| IBIS file stm32u595_599_5a5_5a9_wlcsp150_smps.ibs
[IBIS ver] 4.2
[File name] stm32u595_599_5a5_5a9_wlcsp150_smps.ibs
[File Rev] rev2.0
[Date]  11-09-2023
[Source] Data Created at STMicroelectronics
[Notes]  File originated from ELDO simulations.
[Disclaimer]  This information is for modeling purpose only and is
   not guaranteed. The information is subject to change without
   notice.
[Copyright] Copyright 2023 STMicroelectronics Inc.
|   Component stm32u595_599_5a5_5a9_wlcsp150_smps
[Component] stm32u595_599_5a5_5a9_wlcsp150_smps
[Manufacturer] STMicroelectronics
[Package]
| variable   typ   min   max
R_pkg  0  NA  NA
L_pkg  0  NA  NA
C_pkg  0  NA  NA
[Pin]   signal_name   model_name
A1  VDDUSB  power
A3  VDD  power
A5  PD3  io8_166m_hslv_ft
A7  PG12  io8_100m_hslv_ft
A9  PB5  io8_166m_hslv_ft
A11  VDD11 nc
A13  PE2  io8_100m_hslv_ft
AA1  VSS  gnd
AA3  PB11  io8_100m_hslv_ft
AA5  PE15  io8_100m_hslv_ft
AA7  VSS  gnd
AA9  VSS  gnd
AA11  PA5  io8_100m_ft
AA13  VDDA  nc
AB2  VDD11  nc
AB4  VDDSMPS  nc
AB6  PE14  io8_100m_hslv_ft
AB8  PE7  io8_100m_hslv_ft
AB10  PB2  io8_100m_hslv_tamp_ft
AB12  VDD  power
AC1  VDD  power
AC3  VSSSMPS  nc
AC5  VLXSMPS  nc
AC7  VDD  power
AC9  VDD  power
AC11  PC4  io8_100m_hslv_ft
AC13  VSS  gnd
B2  VDD11  nc
B4  PC11  io8_100m_hslv_ft
B6  VDD  power
B8  VDDIO2  power
B10  PB9  io8_100m_i2c_ft
B12  VDD  power
C1  PA12  io8_100m_ft
C3  VSS  gnd
C5  PD2  io8_100m_ft
C7  PG11  io8_100m_hslv_ft
C9  PB7  io8_spi_hslv_ft
C11  VSS  gnd
C13  VBAT  power
D2  PA13  io8_100m_ft
D4  PC10  io8_100m_ft
D6  VSS  gnd
D8  VSS  gnd
D10  PE3  io8_100m_hslv_tamp_ft
D12  PC13  io8_100m_ft
E1  PA11  io8_100m_ft
E3  PA10  io8_100m_usb_id
E5  PD1  io8_100m_hslv_ft
E7  PG10  io8_100m_hslv_ft
E9  PB6  io8_100m_i2c_ft
E11  PE6  io8_100m_hslv_tamp_ft
E13  PC14-OSC32_IN  nc
F2  PA9  io8_100m_usb_vbus_ft
F4  PA15  nc
F6  PD5  io8_100m_hslv_ft
F8  PG14  io8_100m_hslv_ft
F10  PE4  io8_100m_hslv_tamp_ft
F12  VSS  gnd
G1  PC8  io8_100m_ft
G3  PA8  io8_166m_hslv_ft
G5  PD0  io8_100m_hslv_ft
G7  PG13  io8_100m_hslv_ft
G9  PH3-BOOT0  nc
G11  PF0  io8_100m_hslv_ft
G13  PC15-OSC32_OUT  nc
H2  PC9  io8_100m_ft
H4  PA14  io8_100m_ft
H6  PD4  io8_100m_hslv_ft
H8  PG15  io8_100m_hslv_ft
H10  PE5  io8_100m_hslv_tamp_ft
H12  PF1  io8_100m_hslv_ft
J1  VDDIO2  power
J3  PC6  io8_100m_ft
J5  PC12  io8_166m_hslv_ft
J7  PG9  io8_100m_hslv_ft
J9  PB8  io8_100m_i2c_ft
J11  PF4  io8_spi_ft
J13  PF2  io8_100m_hslv_ft
K2  VSS  gnd
K4  PG8  io8_100m_i2c_ft
K6  PD6  io8_166m_hslv_ft
K8  PB3  io8_100m_i2c_ft
K10  PE1  io8_100m_hslv_ft
K12  PF3  io8_100m_hslv_ft
L1  PG7  io8_100m_hslv_ft
L3  PG5  io8_100m_hslv_ft
L5  PC7  io8_100m_ft
L7  PD7  io8_100m_hslv_ft
L9  PB4  io8_100m_i2c_ft
L11  PF5  io8_spi_ft
L13  VDD  power
M2  PG4  io8_100m_hslv_ft
M4  PG3  io8_100m_hslv_ft
M6  PG6  io8_100m_hslv_ft
M8  PC1  io8_spi_hslv_ft
M10  PE0  io8_100m_hslv_ft
M12  VSS  gnd
N1  PG2  io8_100m_hslv_ft
N3  PD14  io8_100m_hslv_ft
N5  PB15  nc
N7  PC5  io8_100m_tamp_ft
N9  PC0  io8_100m_hslv_ft
N11  PF6  io8_100m_hslv_ft
N13  PF7  io8_100m_hslv_ft
P2  PD15  io8_100m_hslv_ft
P4  PD11  io8_100m_hslv_ft
P6  PF13  io8_100m_hslv_ft
P8  PA4  io8_100m_hslv_ft
P10  PF8  io8_100m_hslv_ft
P12  PF9  io8_100m_hslv_ft
R1  VDD  power
R3  PD12  io8_100m_hslv_ft
R5  PB13  io8_100m_i2c_ft
R7  PF11  io8_166m_hslv_ft
R9  PA2  io8_100m_hslv_ft
R11  PF10  io8_166m_hslv_ft
R13  PH0-OSC_IN   nc
T2  VSS  gnd
T4  PB14  io8_100m_i2c_ft
T6  PG0  io8_100m_hslv_ft
T8  PB0  io8_100m_hslv_ft
T10  PA0  io8_100m_hslv_tamp_ft
T12  NRST  nc
U1  PD13  io8_100m_hslv_ft
U3  PD10  io8_100m_hslv_ft
U5  PE9  io8_166m_hslv_ft
U7  PF14  io8_100m_hslv_ft
U9  PA6  io8_100m_hslv_ft
U11  PC3  io8_100m_hslv_ft
U13  PH1-OSC_OUT  nc
V2  PD9  io8_100m_hslv_ft
V4  PE12  io8_100m_hslv_ft
V6  PE8  io8_100m_hslv_ft
V8  PF12  io8_100m_hslv_ft
V10  PA3  io8_166m_hslv_ft
V12  PC2  io8_100m_hslv_ft
W1  PD8  io8_100m_hslv_ft
W3  PB10  io8_spi_hslv_ft
W5  PE11  io8_100m_hslv_ft
W7  PG1  io8_100m_hslv_ft
W9  PB1  io8_100m_hslv_ft
W11  PA1  io8_100m_hslv_tamp_ft
W13  VSSA_VREFM  nc
Y2  PB12  io8_166m_hslv_ft
Y4  PE13  io8_100m_hslv_ft
Y6  PE10  io8_166m_hslv_ft
Y8  PF15  io8_100m_hslv_ft
Y10  PA7  io8_100m_hslv_ft
Y12  VREFP  nc
[Package Model]   481-wlcsp-150-1rdl-nodsi-220909
[Pin Mapping]   pulldown_ref   pullup_ref   | Comment
A1  nc  vddusb
A3  nc  vddiom
A5  gndio  vddiom
A7  gndio  vddiom  | Depending on IO usage
| A7  gndio  vddio2  | Depending on IO usage
A9  gndio  vddiom
A11  nc  nc
A13  gndio  vddiom
AA1  gndio  nc
AA3  gndio  vddiom
AA5  gndio  vddiom
AA7  gndio  nc
AA9  gndio  nc
AA11  gndio  vddiom
AA13  nc  nc
AB2  nc  nc
AB4  nc  nc
AB6  gndio  vddiom
AB8  gndio  vddiom
AB10  gndio  vddiom
AB12  nc  vddiom
AC1  nc  vddiom
AC3  nc  nc
AC5  nc  nc
AC7  nc  vddiom
AC9  nc  vddiom
AC11  gndio  vddiom
AC13  gndio  nc
B2  nc  nc
B4  gndio  vddiom
B6  nc  vddiom
B8  nc  vddio2
B10  gndio  vddiom
B12  nc  vddiom
C1  gndio  vddiom  | Depending on IO usage
| C1  gndio  vddusb  | Depending on IO usage
C3  gndio  nc
C5  gndio  vddiom
C7  gndio  vddiom  | Depending on IO usage
| C7  gndio  vddio2  | Depending on IO usage
C9  gndio  vddiom
C11  gndio  nc
C13  nc  vsw
D2  gndio  vddiom  | Depending on IO usage
| D2  gndio  vddusb  | Depending on IO usage
D4  gndio  vddiom
D6  gndio  nc
D8  gndio  nc
D10  gndio  vddiom
D12  gndio  vddiom  | Depending on IO usage
| D12  gndio  vsw  | Depending on IO usage
E1  gndio  vddiom  | Depending on IO usage
| E1  gndio  vddusb  | Depending on IO usage
E3  gndio  vddiom  | Depending on IO usage
| E3  gndio  vddusb  | Depending on IO usage
E5  gndio  vddiom
E7  gndio  vddiom  | Depending on IO usage
| E7  gndio  vddio2  | Depending on IO usage
E9  gndio  vddiom
E11  gndio  vddiom
E13  nc  nc
F2  gndio  vddiom  | Depending on IO usage
| F2  gndio  vddusb  | Depending on IO usage
F4  nc  nc
F6  gndio  vddiom
F8  gndio  vddiom  | Depending on IO usage
| F8  gndio  vddio2  | Depending on IO usage
F10  gndio  vddiom
F12  gndio  nc
G1  gndio  vddiom
G3  gndio  vddiom
G5  gndio  vddiom
G7  gndio  vddiom  | Depending on IO usage
| G7  gndio  vddio2  | Depending on IO usage
G9  nc  nc
G11  gndio  vddiom
G13  nc  nc
H2  gndio  vddiom
H4  gndio  vddiom
H6  gndio  vddiom
H8  gndio  vddiom  | Depending on IO usage
| H8  gndio  vddio2  | Depending on IO usage
H10  gndio  vddiom
H12  gndio  vddiom
J1  nc  vddio2
J3  gndio  vddiom
J5  gndio  vddiom
J7  gndio  vddiom  | Depending on IO usage
| J7  gndio  vddio2  | Depending on IO usage
J9  gndio  vddiom
J11  gndio  vddiom
J13  gndio  vddiom
K2  gndio  nc
K4  gndio  vddiom  | Depending on IO usage
| K4  gndio  vddio2  | Depending on IO usage
K6  gndio  vddiom
K8  gndio  vddiom
K10  gndio  vddiom
K12  gndio  vddiom
L1  gndio  vddiom  | Depending on IO usage
| L1  gndio  vddio2  | Depending on IO usage
L3  gndio  vddiom  | Depending on IO usage
| L3  gndio  vddio2  | Depending on IO usage
L5  gndio  vddiom
L7  gndio  vddiom
L9  gndio  vddiom
L11  gndio  vddiom
L13  nc  vddiom
M2  gndio  vddiom  | Depending on IO usage
| M2  gndio  vddio2  | Depending on IO usage
M4  gndio  vddiom  | Depending on IO usage
| M4  gndio  vddio2  | Depending on IO usage
M6  gndio  vddiom  | Depending on IO usage
| M6  gndio  vddio2  | Depending on IO usage
M8  gndio  vddiom
M10  gndio  vddiom
M12  gndio  nc
N1  gndio  vddiom  | Depending on IO usage
| N1  gndio  vddio2  | Depending on IO usage
N3  gndio  vddiom
N5  nc  nc
N7  gndio  vddiom
N9  gndio  vddiom
N11  gndio  vddiom
N13  gndio  vddiom
P2  gndio  vddiom
P4  gndio  vddiom
P6  gndio  vddiom
P8  gndio  vddiom
P10  gndio  vddiom
P12  gndio  vddiom
R1  nc  vddiom
R3  gndio  vddiom
R5  gndio  vddiom
R7  gndio  vddiom
R9  gndio  vddiom
R11  gndio  vddiom
R13  nc  nc
T2  gndio  nc
T4  gndio  vddiom
T6  gndio  vddiom
T8  gndio  vddiom
T10  gndio  vddiom
T12  nc  nc
U1  gndio  vddiom
U3  gndio  vddiom
U5  gndio  vddiom
U7  gndio  vddiom
U9  gndio  vddiom
U11  gndio  vddiom
U13  nc  nc
V2  gndio  vddiom
V4  gndio  vddiom
V6  gndio  vddiom
V8  gndio  vddiom
V10  gndio  vddiom
V12  gndio  vddiom
W1  gndio  vddiom
W3  gndio  vddiom
W5  gndio  vddiom
W7  gndio  vddiom
W9  gndio  vddiom
W11  gndio  vddiom
W13  nc  nc
Y2  gndio  vddiom
Y4  gndio  vddiom
Y6  gndio  vddiom
Y8  gndio  vddiom
Y10  gndio  vddiom
Y12  nc  nc
[Model Selector] io8_100m_ft
io8_100m_ft_hs_1v2  "IO8_FT 100MHz high speed @ 1.2V"
io8_100m_ft_fs_1v2  "IO8_FT 100MHz fast speed @ 1.2V"
io8_100m_ft_fs_pd_1v2  "IO8_FT 100MHz fast speed @ 1.2V pulldown"
io8_100m_ft_ms_1v2  "IO8_FT 100MHz med speed @ 1.2V"
io8_100m_ft_ms_pd_1v2  "IO8_FT 100MHz med speed @ 1.2V pulldown"
io8_100m_ft_ls_1v2  "IO8_FT 100MHz low speed @ 1.2V"
io8_100m_ft_ls_pd_1v2  "IO8_FT 100MHz low speed @ 1.2V pulldown"
io8_100m_ft_hs_1v8  "IO8_FT 100MHz high speed @ 1.8V"
io8_100m_ft_hs_pd_1v8  "IO8_FT 100MHz high speed @ 1.8V pulldown"
io8_100m_ft_fs_1v8  "IO8_FT 100MHz fast speed @ 1.8V"
io8_100m_ft_fs_pd_1v8  "IO8_FT 100MHz fast speed @ 1.8V pulldown"
io8_100m_ft_ms_1v8  "IO8_FT 100MHz med speed @ 1.8V"
io8_100m_ft_ms_pd_1v8  "IO8_FT 100MHz med speed @ 1.8V pulldown"
io8_100m_ft_ls_1v8  "IO8_FT 100MHz low speed @ 1.8V"
io8_100m_ft_ls_pd_1v8  "IO8_FT 100MHz low speed @ 1.8V pulldown"
io8_100m_ft_hs_3v3  "IO8_FT 100MHz high speed @ 3.3V"
io8_100m_ft_hs_pd_3v3  "IO8_FT 100MHz high speed @ 3.3V pulldown"
io8_100m_ft_fs_3v3  "IO8_FT 100MHz fast speed @ 3.3V"
io8_100m_ft_fs_pd_3v3  "IO8_FT 100MHz fast speed @ 3.3V pulldown"
io8_100m_ft_ms_3v3  "IO8_FT 100MHz med speed @ 3.3V"
io8_100m_ft_ms_pd_3v3  "IO8_FT 100MHz med speed @ 3.3V pulldown"
io8_100m_ft_ls_3v3  "IO8_FT 100MHz low speed @ 3.3V"
io8_100m_ft_ls_pd_3v3  "IO8_FT 100MHz low speed @ 3.3V pulldown"
[Model Selector] io8_100m_hslv_ft
io8_100m_ft_hs_1v2  "IO8_FT 100MHz high speed @ 1.2V"
io8_100m_ft_hs_pu_1v2  "IO8_FT 100MHz high speed @ 1.2V pullup"
io8_100m_ft_hs_pd_1v2  "IO8_FT 100MHz high speed @ 1.2V pulldown"
io8_100m_ft_fs_1v2  "IO8_FT 100MHz fast speed @ 1.2V"
io8_100m_ft_fs_pu_1v2  "IO8_FT 100MHz fast speed @ 1.2V pullup"
io8_100m_ft_fs_pd_1v2  "IO8_FT 100MHz fast speed @ 1.2V pulldown"
io8_100m_ft_ms_1v2  "IO8_FT 100MHz med speed @ 1.2V"
io8_100m_ft_ms_pu_1v2  "IO8_FT 100MHz med speed @ 1.2V pullup"
io8_100m_ft_ms_pd_1v2  "IO8_FT 100MHz med speed @ 1.2V pulldown"
io8_100m_ft_ls_1v2  "IO8_FT 100MHz low speed @ 1.2V"
io8_100m_ft_ls_pu_1v2  "IO8_FT 100MHz low speed @ 1.2V pullup"
io8_100m_ft_ls_pd_1v2  "IO8_FT 100MHz low speed @ 1.2V pulldown"
io8_100m_ft_hs_1v8  "IO8_FT 100MHz high speed @ 1.8V"
io8_100m_ft_hs_pu_1v8  "IO8_FT 100MHz high speed @ 1.8V pullup"
io8_100m_ft_hs_pd_1v8  "IO8_FT 100MHz high speed @ 1.8V pulldown"
io8_100m_ft_fs_1v8  "IO8_FT 100MHz fast speed @ 1.8V"
io8_100m_ft_fs_pu_1v8  "IO8_FT 100MHz fast speed @ 1.8V pullup"
io8_100m_ft_fs_pd_1v8  "IO8_FT 100MHz fast speed @ 1.8V pulldown"
io8_100m_ft_ms_1v8  "IO8_FT 100MHz med speed @ 1.8V"
io8_100m_ft_ms_pu_1v8  "IO8_FT 100MHz med speed @ 1.8V pullup"
io8_100m_ft_ms_pd_1v8  "IO8_FT 100MHz med speed @ 1.8V pulldown"
io8_100m_ft_ls_1v8  "IO8_FT 100MHz low speed @ 1.8V"
io8_100m_ft_ls_pu_1v8  "IO8_FT 100MHz low speed @ 1.8V pullup"
io8_100m_ft_ls_pd_1v8  "IO8_FT 100MHz low speed @ 1.8V pulldown"
io8_100m_ft_hs_3v3  "IO8_FT 100MHz high speed @ 3.3V"
io8_100m_ft_hs_pu_3v3  "IO8_FT 100MHz high speed @ 3.3V pullup"
io8_100m_ft_hs_pd_3v3  "IO8_FT 100MHz high speed @ 3.3V pulldown"
io8_100m_ft_fs_3v3  "IO8_FT 100MHz fast speed @ 3.3V"
io8_100m_ft_fs_pu_3v3  "IO8_FT 100MHz fast speed @ 3.3V pullup"
io8_100m_ft_fs_pd_3v3  "IO8_FT 100MHz fast speed @ 3.3V pulldown"
io8_100m_ft_ms_3v3  "IO8_FT 100MHz med speed @ 3.3V"
io8_100m_ft_ms_pu_3v3  "IO8_FT 100MHz med speed @ 3.3V pullup"
io8_100m_ft_ms_pd_3v3  "IO8_FT 100MHz med speed @ 3.3V pulldown"
io8_100m_ft_ls_3v3  "IO8_FT 100MHz low speed @ 3.3V"
io8_100m_ft_ls_pu_3v3  "IO8_FT 100MHz low speed @ 3.3V pullup"
io8_100m_ft_ls_pd_3v3  "IO8_FT 100MHz low speed @ 3.3V pulldown"
io8_100m_hslv_ft_hs_1v2  "IO8_FT 100MHz HSLV high speed @ 1.2V"
io8_100m_hslv_ft_hs_pu_1v2  "IO8_FT 100MHz HSLV high speed @ 1.2V pullup"
io8_100m_hslv_ft_hs_pd_1v2  "IO8_FT 100MHz HSLV high speed @ 1.2V pulldown"
io8_100m_hslv_ft_fs_1v2  "IO8_FT 100MHz HSLV fast speed @ 1.2V"
io8_100m_hslv_ft_fs_pu_1v2  "IO8_FT 100MHz HSLV fast speed @ 1.2V pullup"
io8_100m_hslv_ft_fs_pd_1v2  "IO8_FT 100MHz HSLV fast speed @ 1.2V pulldown"
io8_100m_hslv_ft_ms_1v2  "IO8_FT 100MHz HSLV med speed @ 1.2V"
io8_100m_hslv_ft_ms_pu_1v2  "IO8_FT 100MHz HSLV med speed @ 1.2V pullup"
io8_100m_hslv_ft_ms_pd_1v2  "IO8_FT 100MHz HSLV med speed @ 1.2V pulldown"
io8_100m_hslv_ft_ls_1v2  "IO8_FT 100MHz HSLV low speed @ 1.2V"
io8_100m_hslv_ft_ls_pu_1v2  "IO8_FT 100MHz HSLV low speed @ 1.2V pullup"
io8_100m_hslv_ft_ls_pd_1v2  "IO8_FT 100MHz HSLV low speed @ 1.2V pulldown"
io8_100m_hslv_ft_hs_1v8  "IO8_FT 100MHz HSLV high speed @ 1.8V"
io8_100m_hslv_ft_hs_pu_1v8  "IO8_FT 100MHz HSLV high speed @ 1.8V pullup"
io8_100m_hslv_ft_hs_pd_1v8  "IO8_FT 100MHz HSLV high speed @ 1.8V pulldown"
io8_100m_hslv_ft_fs_1v8  "IO8_FT 100MHz HSLV fast speed @ 1.8V"
io8_100m_hslv_ft_fs_pu_1v8  "IO8_FT 100MHz HSLV fast speed @ 1.8V pullup"
io8_100m_hslv_ft_fs_pd_1v8  "IO8_FT 100MHz HSLV fast speed @ 1.8V pulldown"
io8_100m_hslv_ft_ms_1v8  "IO8_FT 100MHz HSLV med speed @ 1.8V"
io8_100m_hslv_ft_ms_pu_1v8  "IO8_FT 100MHz HSLV med speed @ 1.8V pullup"
io8_100m_hslv_ft_ms_pd_1v8  "IO8_FT 100MHz HSLV med speed @ 1.8V pulldown"
io8_100m_hslv_ft_ls_1v8  "IO8_FT 100MHz HSLV low speed @ 1.8V"
io8_100m_hslv_ft_ls_pu_1v8  "IO8_FT 100MHz HSLV low speed @ 1.8V pullup"
io8_100m_hslv_ft_ls_pd_1v8  "IO8_FT 100MHz HSLV low speed @ 1.8V pulldown"
io8_100m_hslv_ft_hs_2v5  "IO8_FT 100MHz HSLV high speed @ 2.5V"
io8_100m_hslv_ft_hs_pu_2v5  "IO8_FT 100MHz HSLV high speed @ 2.5V pullup"
io8_100m_hslv_ft_hs_pd_2v5  "IO8_FT 100MHz HSLV high speed @ 2.5V pulldown"
io8_100m_hslv_ft_fs_2v5  "IO8_FT 100MHz HSLV fast speed @ 2.5V"
io8_100m_hslv_ft_fs_pu_2v5  "IO8_FT 100MHz HSLV fast speed @ 2.5V pullup"
io8_100m_hslv_ft_fs_pd_2v5  "IO8_FT 100MHz HSLV fast speed @ 2.5V pulldown"
io8_100m_hslv_ft_ms_2v5  "IO8_FT 100MHz HSLV med speed @ 2.5V"
io8_100m_hslv_ft_ms_pu_2v5  "IO8_FT 100MHz HSLV med speed @ 2.5V pullup"
io8_100m_hslv_ft_ms_pd_2v5  "IO8_FT 100MHz HSLV med speed @ 2.5V pulldown"
io8_100m_hslv_ft_ls_2v5  "IO8_FT 100MHz HSLV low speed @ 2.5V"
io8_100m_hslv_ft_ls_pu_2v5  "IO8_FT 100MHz HSLV low speed @ 2.5V pullup"
io8_100m_hslv_ft_ls_pd_2v5  "IO8_FT 100MHz HSLV low speed @ 2.5V pulldown"
[Model Selector] io8_100m_hslv_tamp_ft
io8_100m_ft_hs_1v2  "IO8_FT 100MHz high speed @ 1.2V"
io8_100m_ft_hs_pu_1v2  "IO8_FT 100MHz high speed @ 1.2V pullup"
io8_100m_ft_hs_pd_1v2  "IO8_FT 100MHz high speed @ 1.2V pulldown"
io8_100m_ft_fs_1v2  "IO8_FT 100MHz fast speed @ 1.2V"
io8_100m_ft_fs_pu_1v2  "IO8_FT 100MHz fast speed @ 1.2V pullup"
io8_100m_ft_fs_pd_1v2  "IO8_FT 100MHz fast speed @ 1.2V pulldown"
io8_100m_ft_ms_1v2  "IO8_FT 100MHz med speed @ 1.2V"
io8_100m_ft_ms_pu_1v2  "IO8_FT 100MHz med speed @ 1.2V pullup"
io8_100m_ft_ms_pd_1v2  "IO8_FT 100MHz med speed @ 1.2V pulldown"
io8_100m_ft_ls_1v2  "IO8_FT 100MHz low speed @ 1.2V"
io8_100m_ft_ls_pu_1v2  "IO8_FT 100MHz low speed @ 1.2V pullup"
io8_100m_ft_ls_pd_1v2  "IO8_FT 100MHz low speed @ 1.2V pulldown"
io8_100m_ft_hs_1v8  "IO8_FT 100MHz high speed @ 1.8V"
io8_100m_ft_hs_pu_1v8  "IO8_FT 100MHz high speed @ 1.8V pullup"
io8_100m_ft_hs_pd_1v8  "IO8_FT 100MHz high speed @ 1.8V pulldown"
io8_100m_ft_fs_1v8  "IO8_FT 100MHz fast speed @ 1.8V"
io8_100m_ft_fs_pu_1v8  "IO8_FT 100MHz fast speed @ 1.8V pullup"
io8_100m_ft_fs_pd_1v8  "IO8_FT 100MHz fast speed @ 1.8V pulldown"
io8_100m_ft_ms_1v8  "IO8_FT 100MHz med speed @ 1.8V"
io8_100m_ft_ms_pu_1v8  "IO8_FT 100MHz med speed @ 1.8V pullup"
io8_100m_ft_ms_pd_1v8  "IO8_FT 100MHz med speed @ 1.8V pulldown"
io8_100m_ft_ls_1v8  "IO8_FT 100MHz low speed @ 1.8V"
io8_100m_ft_ls_pu_1v8  "IO8_FT 100MHz low speed @ 1.8V pullup"
io8_100m_ft_ls_pd_1v8  "IO8_FT 100MHz low speed @ 1.8V pulldown"
io8_100m_ft_hs_3v3  "IO8_FT 100MHz high speed @ 3.3V"
io8_100m_ft_hs_pu_3v3  "IO8_FT 100MHz high speed @ 3.3V pullup"
io8_100m_ft_hs_pd_3v3  "IO8_FT 100MHz high speed @ 3.3V pulldown"
io8_100m_ft_fs_3v3  "IO8_FT 100MHz fast speed @ 3.3V"
io8_100m_ft_fs_pu_3v3  "IO8_FT 100MHz fast speed @ 3.3V pullup"
io8_100m_ft_fs_pd_3v3  "IO8_FT 100MHz fast speed @ 3.3V pulldown"
io8_100m_ft_ms_3v3  "IO8_FT 100MHz med speed @ 3.3V"
io8_100m_ft_ms_pu_3v3  "IO8_FT 100MHz med speed @ 3.3V pullup"
io8_100m_ft_ms_pd_3v3  "IO8_FT 100MHz med speed @ 3.3V pulldown"
io8_100m_ft_ls_3v3  "IO8_FT 100MHz low speed @ 3.3V"
io8_100m_ft_ls_pu_3v3  "IO8_FT 100MHz low speed @ 3.3V pullup"
io8_100m_ft_ls_pd_3v3  "IO8_FT 100MHz low speed @ 3.3V pulldown"
io8_100m_hslv_ft_hs_1v2  "IO8_FT 100MHz HSLV high speed @ 1.2V"
io8_100m_hslv_ft_hs_pu_1v2  "IO8_FT 100MHz HSLV high speed @ 1.2V pullup"
io8_100m_hslv_ft_hs_pd_1v2  "IO8_FT 100MHz HSLV high speed @ 1.2V pulldown"
io8_100m_hslv_ft_fs_1v2  "IO8_FT 100MHz HSLV fast speed @ 1.2V"
io8_100m_hslv_ft_fs_pu_1v2  "IO8_FT 100MHz HSLV fast speed @ 1.2V pullup"
io8_100m_hslv_ft_fs_pd_1v2  "IO8_FT 100MHz HSLV fast speed @ 1.2V pulldown"
io8_100m_hslv_ft_ms_1v2  "IO8_FT 100MHz HSLV med speed @ 1.2V"
io8_100m_hslv_ft_ms_pu_1v2  "IO8_FT 100MHz HSLV med speed @ 1.2V pullup"
io8_100m_hslv_ft_ms_pd_1v2  "IO8_FT 100MHz HSLV med speed @ 1.2V pulldown"
io8_100m_hslv_ft_ls_1v2  "IO8_FT 100MHz HSLV low speed @ 1.2V"
io8_100m_hslv_ft_ls_pu_1v2  "IO8_FT 100MHz HSLV low speed @ 1.2V pullup"
io8_100m_hslv_ft_ls_pd_1v2  "IO8_FT 100MHz HSLV low speed @ 1.2V pulldown"
io8_100m_hslv_ft_hs_1v8  "IO8_FT 100MHz HSLV high speed @ 1.8V"
io8_100m_hslv_ft_hs_pu_1v8  "IO8_FT 100MHz HSLV high speed @ 1.8V pullup"
io8_100m_hslv_ft_hs_pd_1v8  "IO8_FT 100MHz HSLV high speed @ 1.8V pulldown"
io8_100m_hslv_ft_fs_1v8  "IO8_FT 100MHz HSLV fast speed @ 1.8V"
io8_100m_hslv_ft_fs_pu_1v8  "IO8_FT 100MHz HSLV fast speed @ 1.8V pullup"
io8_100m_hslv_ft_fs_pd_1v8  "IO8_FT 100MHz HSLV fast speed @ 1.8V pulldown"
io8_100m_hslv_ft_ms_1v8  "IO8_FT 100MHz HSLV med speed @ 1.8V"
io8_100m_hslv_ft_ms_pu_1v8  "IO8_FT 100MHz HSLV med speed @ 1.8V pullup"
io8_100m_hslv_ft_ms_pd_1v8  "IO8_FT 100MHz HSLV med speed @ 1.8V pulldown"
io8_100m_hslv_ft_ls_1v8  "IO8_FT 100MHz HSLV low speed @ 1.8V"
io8_100m_hslv_ft_ls_pu_1v8  "IO8_FT 100MHz HSLV low speed @ 1.8V pullup"
io8_100m_hslv_ft_ls_pd_1v8  "IO8_FT 100MHz HSLV low speed @ 1.8V pulldown"
io8_100m_hslv_ft_hs_2v5  "IO8_FT 100MHz HSLV high speed @ 2.5V"
io8_100m_hslv_ft_hs_pu_2v5  "IO8_FT 100MHz HSLV high speed @ 2.5V pullup"
io8_100m_hslv_ft_hs_pd_2v5  "IO8_FT 100MHz HSLV high speed @ 2.5V pulldown"
io8_100m_hslv_ft_fs_2v5  "IO8_FT 100MHz HSLV fast speed @ 2.5V"
io8_100m_hslv_ft_fs_pu_2v5  "IO8_FT 100MHz HSLV fast speed @ 2.5V pullup"
io8_100m_hslv_ft_fs_pd_2v5  "IO8_FT 100MHz HSLV fast speed @ 2.5V pulldown"
io8_100m_hslv_ft_ms_2v5  "IO8_FT 100MHz HSLV med speed @ 2.5V"
io8_100m_hslv_ft_ms_pu_2v5  "IO8_FT 100MHz HSLV med speed @ 2.5V pullup"
io8_100m_hslv_ft_ms_pd_2v5  "IO8_FT 100MHz HSLV med speed @ 2.5V pulldown"
io8_100m_hslv_ft_ls_2v5  "IO8_FT 100MHz HSLV low speed @ 2.5V"
io8_100m_hslv_ft_ls_pu_2v5  "IO8_FT 100MHz HSLV low speed @ 2.5V pullup"
io8_100m_hslv_ft_ls_pd_2v5  "IO8_FT 100MHz HSLV low speed @ 2.5V pulldown"
io8_ft_v33_hs_1v2  "IO8_FT_V33 high speed @ 1.2V"
io8_ft_v33_hs_pu_1v2  "IO8_FT_V33 high speed @ 1.2V pullup"
io8_ft_v33_hs_pd_1v2  "IO8_FT_V33 high speed @ 1.2V pulldown"
io8_ft_v33_fs_1v2  "IO8_FT_V33 fast speed @ 1.2V"
io8_ft_v33_fs_pu_1v2  "IO8_FT_V33 fast speed @ 1.2V pullup"
io8_ft_v33_fs_pd_1v2  "IO8_FT_V33 fast speed @ 1.2V pulldown"
io8_ft_v33_ms_1v2  "IO8_FT_V33 med speed @ 1.2V"
io8_ft_v33_ms_pu_1v2  "IO8_FT_V33 med speed @ 1.2V pullup"
io8_ft_v33_ms_pd_1v2  "IO8_FT_V33 med speed @ 1.2V pulldown"
io8_ft_v33_ls_1v2  "IO8_FT_V33 low speed @ 1.2V"
io8_ft_v33_ls_pu_1v2  "IO8_FT_V33 low speed @ 1.2V pullup"
io8_ft_v33_ls_pd_1v2  "IO8_FT_V33 low speed @ 1.2V pulldown"
io8_ft_v33_hs_1v8  "IO8_FT_V33 high speed @ 1.8V"
io8_ft_v33_hs_pu_1v8  "IO8_FT_V33 high speed @ 1.8V pullup"
io8_ft_v33_hs_pd_1v8  "IO8_FT_V33 high speed @ 1.8V pulldown"
io8_ft_v33_fs_1v8  "IO8_FT_V33 fast speed @ 1.8V"
io8_ft_v33_fs_pu_1v8  "IO8_FT_V33 fast speed @ 1.8V pullup"
io8_ft_v33_fs_pd_1v8  "IO8_FT_V33 fast speed @ 1.8V pulldown"
io8_ft_v33_ms_1v8  "IO8_FT_V33 med speed @ 1.8V"
io8_ft_v33_ms_pu_1v8  "IO8_FT_V33 med speed @ 1.8V pullup"
io8_ft_v33_ms_pd_1v8  "IO8_FT_V33 med speed @ 1.8V pulldown"
io8_ft_v33_ls_1v8  "IO8_FT_V33 low speed @ 1.8V"
io8_ft_v33_ls_pu_1v8  "IO8_FT_V33 low speed @ 1.8V pullup"
io8_ft_v33_ls_pd_1v8  "IO8_FT_V33 low speed @ 1.8V pulldown"
io8_ft_v33_hs_3v3  "IO8_FT_V33 high speed @ 3.3V"
io8_ft_v33_hs_pu_3v3  "IO8_FT_V33 high speed @ 3.3V pullup"
io8_ft_v33_hs_pd_3v3  "IO8_FT_V33 high speed @ 3.3V pulldown"
io8_ft_v33_fs_3v3  "IO8_FT_V33 fast speed @ 3.3V"
io8_ft_v33_fs_pu_3v3  "IO8_FT_V33 fast speed @ 3.3V pullup"
io8_ft_v33_fs_pd_3v3  "IO8_FT_V33 fast speed @ 3.3V pulldown"
io8_ft_v33_ms_3v3  "IO8_FT_V33 med speed @ 3.3V"
io8_ft_v33_ms_pu_3v3  "IO8_FT_V33 med speed @ 3.3V pullup"
io8_ft_v33_ms_pd_3v3  "IO8_FT_V33 med speed @ 3.3V pulldown"
io8_ft_v33_ls_3v3  "IO8_FT_V33 low speed @ 3.3V"
io8_ft_v33_ls_pu_3v3  "IO8_FT_V33 low speed @ 3.3V pullup"
io8_ft_v33_ls_pd_3v3  "IO8_FT_V33 low speed @ 3.3V pulldown"
[Model Selector] io8_100m_i2c_ft
io8_100m_ft_hs_1v2  "IO8_FT 100MHz high speed @ 1.2V"
io8_100m_ft_hs_pu_1v2  "IO8_FT 100MHz high speed @ 1.2V pullup"
io8_100m_ft_hs_pd_1v2  "IO8_FT 100MHz high speed @ 1.2V pulldown"
io8_100m_ft_fs_1v2  "IO8_FT 100MHz fast speed @ 1.2V"
io8_100m_ft_fs_pu_1v2  "IO8_FT 100MHz fast speed @ 1.2V pullup"
io8_100m_ft_fs_pd_1v2  "IO8_FT 100MHz fast speed @ 1.2V pulldown"
io8_100m_ft_ms_1v2  "IO8_FT 100MHz med speed @ 1.2V"
io8_100m_ft_ms_pu_1v2  "IO8_FT 100MHz med speed @ 1.2V pullup"
io8_100m_ft_ms_pd_1v2  "IO8_FT 100MHz med speed @ 1.2V pulldown"
io8_100m_ft_ls_1v2  "IO8_FT 100MHz low speed @ 1.2V"
io8_100m_ft_ls_pu_1v2  "IO8_FT 100MHz low speed @ 1.2V pullup"
io8_100m_ft_ls_pd_1v2  "IO8_FT 100MHz low speed @ 1.2V pulldown"
io8_100m_ft_hs_1v8  "IO8_FT 100MHz high speed @ 1.8V"
io8_100m_ft_hs_pu_1v8  "IO8_FT 100MHz high speed @ 1.8V pullup"
io8_100m_ft_hs_pd_1v8  "IO8_FT 100MHz high speed @ 1.8V pulldown"
io8_100m_ft_fs_1v8  "IO8_FT 100MHz fast speed @ 1.8V"
io8_100m_ft_fs_pu_1v8  "IO8_FT 100MHz fast speed @ 1.8V pullup"
io8_100m_ft_fs_pd_1v8  "IO8_FT 100MHz fast speed @ 1.8V pulldown"
io8_100m_ft_ms_1v8  "IO8_FT 100MHz med speed @ 1.8V"
io8_100m_ft_ms_pu_1v8  "IO8_FT 100MHz med speed @ 1.8V pullup"
io8_100m_ft_ms_pd_1v8  "IO8_FT 100MHz med speed @ 1.8V pulldown"
io8_100m_ft_ls_1v8  "IO8_FT 100MHz low speed @ 1.8V"
io8_100m_ft_ls_pu_1v8  "IO8_FT 100MHz low speed @ 1.8V pullup"
io8_100m_ft_ls_pd_1v8  "IO8_FT 100MHz low speed @ 1.8V pulldown"
io8_100m_ft_hs_3v3  "IO8_FT 100MHz high speed @ 3.3V"
io8_100m_ft_hs_pu_3v3  "IO8_FT 100MHz high speed @ 3.3V pullup"
io8_100m_ft_hs_pd_3v3  "IO8_FT 100MHz high speed @ 3.3V pulldown"
io8_100m_ft_fs_3v3  "IO8_FT 100MHz fast speed @ 3.3V"
io8_100m_ft_fs_pu_3v3  "IO8_FT 100MHz fast speed @ 3.3V pullup"
io8_100m_ft_fs_pd_3v3  "IO8_FT 100MHz fast speed @ 3.3V pulldown"
io8_100m_ft_ms_3v3  "IO8_FT 100MHz med speed @ 3.3V"
io8_100m_ft_ms_pu_3v3  "IO8_FT 100MHz med speed @ 3.3V pullup"
io8_100m_ft_ms_pd_3v3  "IO8_FT 100MHz med speed @ 3.3V pulldown"
io8_100m_ft_ls_3v3  "IO8_FT 100MHz low speed @ 3.3V"
io8_100m_ft_ls_pu_3v3  "IO8_FT 100MHz low speed @ 3.3V pullup"
io8_100m_ft_ls_pd_3v3  "IO8_FT 100MHz low speed @ 3.3V pulldown"
io8_100m_i2c_ft_1v2  "IO8_FT 100MHz I2C @ 1.2V"
io8_100m_i2c_ft_pu_1v2  "IO8_FT 100MHz I2C @ 1.2V pullup"
io8_100m_i2c_ft_pd_1v2  "IO8_FT 100MHz I2C @ 1.2V pulldown"
io8_100m_i2c_ft_1v8  "IO8_FT 100MHz I2C @ 1.8V"
io8_100m_i2c_ft_pu_1v8  "IO8_FT 100MHz I2C @ 1.8V pullup"
io8_100m_i2c_ft_pd_1v8  "IO8_FT 100MHz I2C @ 1,8V pulldown"
io8_100m_i2c_ft_3v3  "IO8_FT 100MHz I2C @ 3.3V"
io8_100m_i2c_ft_pu_3v3  "IO8_FT 100MHz I2C HSLV @ 3.3V pullup"
io8_100m_i2c_ft_pd_3v3  "IO8_FT 100MHz I2C @ 3.3V pulldown"
[Model Selector] io8_100m_tamp_ft
io8_100m_ft_hs_1v2  "IO8_FT 100MHz high speed @ 1.2V"
io8_100m_ft_hs_pu_1v2  "IO8_FT 100MHz high speed @ 1.2V pullup"
io8_100m_ft_hs_pd_1v2  "IO8_FT 100MHz high speed @ 1.2V pulldown"
io8_100m_ft_fs_1v2  "IO8_FT 100MHz fast speed @ 1.2V"
io8_100m_ft_fs_pu_1v2  "IO8_FT 100MHz fast speed @ 1.2V pullup"
io8_100m_ft_fs_pd_1v2  "IO8_FT 100MHz fast speed @ 1.2V pulldown"
io8_100m_ft_ms_1v2  "IO8_FT 100MHz med speed @ 1.2V"
io8_100m_ft_ms_pu_1v2  "IO8_FT 100MHz med speed @ 1.2V pullup"
io8_100m_ft_ms_pd_1v2  "IO8_FT 100MHz med speed @ 1.2V pulldown"
io8_100m_ft_ls_1v2  "IO8_FT 100MHz low speed @ 1.2V"
io8_100m_ft_ls_pu_1v2  "IO8_FT 100MHz low speed @ 1.2V pullup"
io8_100m_ft_ls_pd_1v2  "IO8_FT 100MHz low speed @ 1.2V pulldown"
io8_100m_ft_hs_1v8  "IO8_FT 100MHz high speed @ 1.8V"
io8_100m_ft_hs_pu_1v8  "IO8_FT 100MHz high speed @ 1.8V pullup"
io8_100m_ft_hs_pd_1v8  "IO8_FT 100MHz high speed @ 1.8V pulldown"
io8_100m_ft_fs_1v8  "IO8_FT 100MHz fast speed @ 1.8V"
io8_100m_ft_fs_pu_1v8  "IO8_FT 100MHz fast speed @ 1.8V pullup"
io8_100m_ft_fs_pd_1v8  "IO8_FT 100MHz fast speed @ 1.8V pulldown"
io8_100m_ft_ms_1v8  "IO8_FT 100MHz med speed @ 1.8V"
io8_100m_ft_ms_pu_1v8  "IO8_FT 100MHz med speed @ 1.8V pullup"
io8_100m_ft_ms_pd_1v8  "IO8_FT 100MHz med speed @ 1.8V pulldown"
io8_100m_ft_ls_1v8  "IO8_FT 100MHz low speed @ 1.8V"
io8_100m_ft_ls_pu_1v8  "IO8_FT 100MHz low speed @ 1.8V pullup"
io8_100m_ft_ls_pd_1v8  "IO8_FT 100MHz low speed @ 1.8V pulldown"
io8_100m_ft_hs_3v3  "IO8_FT 100MHz high speed @ 3.3V"
io8_100m_ft_hs_pu_3v3  "IO8_FT 100MHz high speed @ 3.3V pullup"
io8_100m_ft_hs_pd_3v3  "IO8_FT 100MHz high speed @ 3.3V pulldown"
io8_100m_ft_fs_3v3  "IO8_FT 100MHz fast speed @ 3.3V"
io8_100m_ft_fs_pu_3v3  "IO8_FT 100MHz fast speed @ 3.3V pullup"
io8_100m_ft_fs_pd_3v3  "IO8_FT 100MHz fast speed @ 3.3V pulldown"
io8_100m_ft_ms_3v3  "IO8_FT 100MHz med speed @ 3.3V"
io8_100m_ft_ms_pu_3v3  "IO8_FT 100MHz med speed @ 3.3V pullup"
io8_100m_ft_ms_pd_3v3  "IO8_FT 100MHz med speed @ 3.3V pulldown"
io8_100m_ft_ls_3v3  "IO8_FT 100MHz low speed @ 3.3V"
io8_100m_ft_ls_pu_3v3  "IO8_FT 100MHz low speed @ 3.3V pullup"
io8_100m_ft_ls_pd_3v3  "IO8_FT 100MHz low speed @ 3.3V pulldown"
io8_ft_v33_hs_1v2  "IO8_FT_V33 high speed @ 1.2V"
io8_ft_v33_hs_pu_1v2  "IO8_FT_V33 high speed @ 1.2V pullup"
io8_ft_v33_hs_pd_1v2  "IO8_FT_V33 high speed @ 1.2V pulldown"
io8_ft_v33_fs_1v2  "IO8_FT_V33 fast speed @ 1.2V"
io8_ft_v33_fs_pu_1v2  "IO8_FT_V33 fast speed @ 1.2V pullup"
io8_ft_v33_fs_pd_1v2  "IO8_FT_V33 fast speed @ 1.2V pulldown"
io8_ft_v33_ms_1v2  "IO8_FT_V33 med speed @ 1.2V"
io8_ft_v33_ms_pu_1v2  "IO8_FT_V33 med speed @ 1.2V pullup"
io8_ft_v33_ms_pd_1v2  "IO8_FT_V33 med speed @ 1.2V pulldown"
io8_ft_v33_ls_1v2  "IO8_FT_V33 low speed @ 1.2V"
io8_ft_v33_ls_pu_1v2  "IO8_FT_V33 low speed @ 1.2V pullup"
io8_ft_v33_ls_pd_1v2  "IO8_FT_V33 low speed @ 1.2V pulldown"
io8_ft_v33_hs_1v8  "IO8_FT_V33 high speed @ 1.8V"
io8_ft_v33_hs_pu_1v8  "IO8_FT_V33 high speed @ 1.8V pullup"
io8_ft_v33_hs_pd_1v8  "IO8_FT_V33 high speed @ 1.8V pulldown"
io8_ft_v33_fs_1v8  "IO8_FT_V33 fast speed @ 1.8V"
io8_ft_v33_fs_pu_1v8  "IO8_FT_V33 fast speed @ 1.8V pullup"
io8_ft_v33_fs_pd_1v8  "IO8_FT_V33 fast speed @ 1.8V pulldown"
io8_ft_v33_ms_1v8  "IO8_FT_V33 med speed @ 1.8V"
io8_ft_v33_ms_pu_1v8  "IO8_FT_V33 med speed @ 1.8V pullup"
io8_ft_v33_ms_pd_1v8  "IO8_FT_V33 med speed @ 1.8V pulldown"
io8_ft_v33_ls_1v8  "IO8_FT_V33 low speed @ 1.8V"
io8_ft_v33_ls_pu_1v8  "IO8_FT_V33 low speed @ 1.8V pullup"
io8_ft_v33_ls_pd_1v8  "IO8_FT_V33 low speed @ 1.8V pulldown"
io8_ft_v33_hs_3v3  "IO8_FT_V33 high speed @ 3.3V"
io8_ft_v33_hs_pu_3v3  "IO8_FT_V33 high speed @ 3.3V pullup"
io8_ft_v33_hs_pd_3v3  "IO8_FT_V33 high speed @ 3.3V pulldown"
io8_ft_v33_fs_3v3  "IO8_FT_V33 fast speed @ 3.3V"
io8_ft_v33_fs_pu_3v3  "IO8_FT_V33 fast speed @ 3.3V pullup"
io8_ft_v33_fs_pd_3v3  "IO8_FT_V33 fast speed @ 3.3V pulldown"
io8_ft_v33_ms_3v3  "IO8_FT_V33 med speed @ 3.3V"
io8_ft_v33_ms_pu_3v3  "IO8_FT_V33 med speed @ 3.3V pullup"
io8_ft_v33_ms_pd_3v3  "IO8_FT_V33 med speed @ 3.3V pulldown"
io8_ft_v33_ls_3v3  "IO8_FT_V33 low speed @ 3.3V"
io8_ft_v33_ls_pu_3v3  "IO8_FT_V33 low speed @ 3.3V pullup"
io8_ft_v33_ls_pd_3v3  "IO8_FT_V33 low speed @ 3.3V pulldown"
[Model Selector] io8_100m_usb_id
io8_100m_ft_hs_1v2  "IO8_FT 100MHz high speed @ 1.2V"
io8_100m_ft_hs_pu_1v2  "IO8_FT 100MHz high speed @ 1.2V pullup"
io8_100m_ft_hs_pd_1v2  "IO8_FT 100MHz high speed @ 1.2V pulldown"
io8_100m_ft_fs_1v2  "IO8_FT 100MHz fast speed @ 1.2V"
io8_100m_ft_fs_pu_1v2  "IO8_FT 100MHz fast speed @ 1.2V pullup"
io8_100m_ft_fs_pd_1v2  "IO8_FT 100MHz fast speed @ 1.2V pulldown"
io8_100m_ft_ms_1v2  "IO8_FT 100MHz med speed @ 1.2V"
io8_100m_ft_ms_pu_1v2  "IO8_FT 100MHz med speed @ 1.2V pullup"
io8_100m_ft_ms_pd_1v2  "IO8_FT 100MHz med speed @ 1.2V pulldown"
io8_100m_ft_ls_1v2  "IO8_FT 100MHz low speed @ 1.2V"
io8_100m_ft_ls_pu_1v2  "IO8_FT 100MHz low speed @ 1.2V pullup"
io8_100m_ft_ls_pd_1v2  "IO8_FT 100MHz low speed @ 1.2V pulldown"
io8_100m_ft_hs_1v8  "IO8_FT 100MHz high speed @ 1.8V"
io8_100m_ft_hs_pu_1v8  "IO8_FT 100MHz high speed @ 1.8V pullup"
io8_100m_ft_hs_pd_1v8  "IO8_FT 100MHz high speed @ 1.8V pulldown"
io8_100m_ft_fs_1v8  "IO8_FT 100MHz fast speed @ 1.8V"
io8_100m_ft_fs_pu_1v8  "IO8_FT 100MHz fast speed @ 1.8V pullup"
io8_100m_ft_fs_pd_1v8  "IO8_FT 100MHz fast speed @ 1.8V pulldown"
io8_100m_ft_ms_1v8  "IO8_FT 100MHz med speed @ 1.8V"
io8_100m_ft_ms_pu_1v8  "IO8_FT 100MHz med speed @ 1.8V pullup"
io8_100m_ft_ms_pd_1v8  "IO8_FT 100MHz med speed @ 1.8V pulldown"
io8_100m_ft_ls_1v8  "IO8_FT 100MHz low speed @ 1.8V"
io8_100m_ft_ls_pu_1v8  "IO8_FT 100MHz low speed @ 1.8V pullup"
io8_100m_ft_ls_pd_1v8  "IO8_FT 100MHz low speed @ 1.8V pulldown"
io8_100m_ft_hs_3v3  "IO8_FT 100MHz high speed @ 3.3V"
io8_100m_ft_hs_pu_3v3  "IO8_FT 100MHz high speed @ 3.3V pullup"
io8_100m_ft_hs_pd_3v3  "IO8_FT 100MHz high speed @ 3.3V pulldown"
io8_100m_ft_fs_3v3  "IO8_FT 100MHz fast speed @ 3.3V"
io8_100m_ft_fs_pu_3v3  "IO8_FT 100MHz fast speed @ 3.3V pullup"
io8_100m_ft_fs_pd_3v3  "IO8_FT 100MHz fast speed @ 3.3V pulldown"
io8_100m_ft_ms_3v3  "IO8_FT 100MHz med speed @ 3.3V"
io8_100m_ft_ms_pu_3v3  "IO8_FT 100MHz med speed @ 3.3V pullup"
io8_100m_ft_ms_pd_3v3  "IO8_FT 100MHz med speed @ 3.3V pulldown"
io8_100m_ft_ls_3v3  "IO8_FT 100MHz low speed @ 3.3V"
io8_100m_ft_ls_pu_3v3  "IO8_FT 100MHz low speed @ 3.3V pullup"
io8_100m_ft_ls_pd_3v3  "IO8_FT 100MHz low speed @ 3.3V pulldown"
io8usb_id_nopu  "IOUSB ID @ 3.3V"
io8usb_id_pu  "IOUSB ID @ 3.3V pullup"
[Model Selector] io8_100m_usb_vbus_ft
io8_100m_ft_hs_1v2  "IO8_FT 100MHz high speed @ 1.2V"
io8_100m_ft_hs_pu_1v2  "IO8_FT 100MHz high speed @ 1.2V pullup"
io8_100m_ft_hs_pd_1v2  "IO8_FT 100MHz high speed @ 1.2V pulldown"
io8_100m_ft_fs_1v2  "IO8_FT 100MHz fast speed @ 1.2V"
io8_100m_ft_fs_pu_1v2  "IO8_FT 100MHz fast speed @ 1.2V pullup"
io8_100m_ft_fs_pd_1v2  "IO8_FT 100MHz fast speed @ 1.2V pulldown"
io8_100m_ft_ms_1v2  "IO8_FT 100MHz med speed @ 1.2V"
io8_100m_ft_ms_pu_1v2  "IO8_FT 100MHz med speed @ 1.2V pullup"
io8_100m_ft_ms_pd_1v2  "IO8_FT 100MHz med speed @ 1.2V pulldown"
io8_100m_ft_ls_1v2  "IO8_FT 100MHz low speed @ 1.2V"
io8_100m_ft_ls_pu_1v2  "IO8_FT 100MHz low speed @ 1.2V pullup"
io8_100m_ft_ls_pd_1v2  "IO8_FT 100MHz low speed @ 1.2V pulldown"
io8_100m_ft_hs_1v8  "IO8_FT 100MHz high speed @ 1.8V"
io8_100m_ft_hs_pu_1v8  "IO8_FT 100MHz high speed @ 1.8V pullup"
io8_100m_ft_hs_pd_1v8  "IO8_FT 100MHz high speed @ 1.8V pulldown"
io8_100m_ft_fs_1v8  "IO8_FT 100MHz fast speed @ 1.8V"
io8_100m_ft_fs_pu_1v8  "IO8_FT 100MHz fast speed @ 1.8V pullup"
io8_100m_ft_fs_pd_1v8  "IO8_FT 100MHz fast speed @ 1.8V pulldown"
io8_100m_ft_ms_1v8  "IO8_FT 100MHz med speed @ 1.8V"
io8_100m_ft_ms_pu_1v8  "IO8_FT 100MHz med speed @ 1.8V pullup"
io8_100m_ft_ms_pd_1v8  "IO8_FT 100MHz med speed @ 1.8V pulldown"
io8_100m_ft_ls_1v8  "IO8_FT 100MHz low speed @ 1.8V"
io8_100m_ft_ls_pu_1v8  "IO8_FT 100MHz low speed @ 1.8V pullup"
io8_100m_ft_ls_pd_1v8  "IO8_FT 100MHz low speed @ 1.8V pulldown"
io8_100m_ft_hs_3v3  "IO8_FT 100MHz high speed @ 3.3V"
io8_100m_ft_hs_pu_3v3  "IO8_FT 100MHz high speed @ 3.3V pullup"
io8_100m_ft_hs_pd_3v3  "IO8_FT 100MHz high speed @ 3.3V pulldown"
io8_100m_ft_fs_3v3  "IO8_FT 100MHz fast speed @ 3.3V"
io8_100m_ft_fs_pu_3v3  "IO8_FT 100MHz fast speed @ 3.3V pullup"
io8_100m_ft_fs_pd_3v3  "IO8_FT 100MHz fast speed @ 3.3V pulldown"
io8_100m_ft_ms_3v3  "IO8_FT 100MHz med speed @ 3.3V"
io8_100m_ft_ms_pu_3v3  "IO8_FT 100MHz med speed @ 3.3V pullup"
io8_100m_ft_ms_pd_3v3  "IO8_FT 100MHz med speed @ 3.3V pulldown"
io8_100m_ft_ls_3v3  "IO8_FT 100MHz low speed @ 3.3V"
io8_100m_ft_ls_pu_3v3  "IO8_FT 100MHz low speed @ 3.3V pullup"
io8_100m_ft_ls_pd_3v3  "IO8_FT 100MHz low speed @ 3.3V pulldown"
io8usb_adp "IOUSB ADP @ 3.3V"
io8usb_vbus "IOUSB VBUS @ 3.3V"
[Model Selector] io8_166m_hslv_ft
io8_166m_ft_hs_1v2  "IO8_FT 166MHz high speed @ 1.2V"
io8_166m_ft_hs_pu_1v2  "IO8_FT 166MHz high speed @ 1.2V pullup"
io8_166m_ft_hs_pd_1v2  "IO8_FT 166MHz high speed @ 1.2V pulldown"
io8_166m_ft_fs_1v2  "IO8_FT 166MHz fast speed @ 1.2V"
io8_166m_ft_fs_pu_1v2  "IO8_FT 166MHz fast speed @ 1.2V pullup"
io8_166m_ft_fs_pd_1v2  "IO8_FT 166MHz fast speed @ 1.2V pulldown"
io8_166m_ft_ms_1v2  "IO8_FT 166MHz med speed @ 1.2V"
io8_166m_ft_ms_pu_1v2  "IO8_FT 166MHz med speed @ 1.2V pullup"
io8_166m_ft_ms_pd_1v2  "IO8_FT 166MHz med speed @ 1.2V pulldown"
io8_166m_ft_ls_1v2  "IO8_FT 166MHz low speed @ 1.2V"
io8_166m_ft_ls_pu_1v2  "IO8_FT 166MHz low speed @ 1.2V pullup"
io8_166m_ft_ls_pd_1v2  "IO8_FT 166MHz low speed @ 1.2V pulldown"
io8_166m_ft_hs_1v8  "IO8_FT 166MHz high speed @ 1.8V"
io8_166m_ft_hs_pu_1v8  "IO8_FT 166MHz high speed @ 1.8V pullup"
io8_166m_ft_hs_pd_1v8  "IO8_FT 166MHz high speed @ 1.8V pulldown"
io8_166m_ft_fs_1v8  "IO8_FT 166MHz fast speed @ 1.8V"
io8_166m_ft_fs_pu_1v8  "IO8_FT 166MHz fast speed @ 1.8V pullup"
io8_166m_ft_fs_pd_1v8  "IO8_FT 166MHz fast speed @ 1.8V pulldown"
io8_166m_ft_ms_1v8  "IO8_FT 166MHz med speed @ 1.8V"
io8_166m_ft_ms_pu_1v8  "IO8_FT 166MHz med speed @ 1.8V pullup"
io8_166m_ft_ms_pd_1v8  "IO8_FT 166MHz med speed @ 1.8V pulldown"
io8_166m_ft_ls_1v8  "IO8_FT 166MHz low speed @ 1.8V"
io8_166m_ft_ls_pu_1v8  "IO8_FT 166MHz low speed @ 1.8V pullup"
io8_166m_ft_ls_pd_1v8  "IO8_FT 166MHz low speed @ 1.8V pulldown"
io8_166m_ft_hs_3v3  "IO8_FT 166MHz high speed @ 3.3V"
io8_166m_ft_hs_pu_3v3  "IO8_FT 166MHz high speed @ 3.3V pullup"
io8_166m_ft_hs_pd_3v3  "IO8_FT 166MHz high speed @ 3.3V pulldown"
io8_166m_ft_fs_3v3  "IO8_FT 166MHz fast speed @ 3.3V"
io8_166m_ft_fs_pu_3v3  "IO8_FT 166MHz fast speed @ 3.3V pullup"
io8_166m_ft_fs_pd_3v3  "IO8_FT 166MHz fast speed @ 3.3V pulldown"
io8_166m_ft_ms_3v3  "IO8_FT 166MHz med speed @ 3.3V"
io8_166m_ft_ms_pu_3v3  "IO8_FT 166MHz med speed @ 3.3V pullup"
io8_166m_ft_ms_pd_3v3  "IO8_FT 166MHz med speed @ 3.3V pulldown"
io8_166m_ft_ls_3v3  "IO8_FT 166MHz low speed @ 3.3V"
io8_166m_ft_ls_pu_3v3  "IO8_FT 166MHz low speed @ 3.3V pullup"
io8_166m_ft_ls_pd_3v3  "IO8_FT 166MHz low speed @ 3.3V pulldown"
io8_166m_hslv_ft_hs_1v2  "IO8_FT 166MHz HSLV high speed @ 1.2V"
io8_166m_hslv_ft_hs_pu_1v2  "IO8_FT 166MHz HSLV high speed @ 1.2V pullup"
io8_166m_hslv_ft_hs_pd_1v2  "IO8_FT 166MHz HSLV high speed @ 1.2V pulldown"
io8_166m_hslv_ft_fs_1v2  "IO8_FT 166MHz HSLV fast speed @ 1.2V"
io8_166m_hslv_ft_fs_pu_1v2  "IO8_FT 166MHz HSLV fast speed @ 1.2V pullup"
io8_166m_hslv_ft_fs_pd_1v2  "IO8_FT 166MHz HSLV fast speed @ 1.2V pulldown"
io8_166m_hslv_ft_ms_1v2  "IO8_FT 166MHz HSLV med speed @ 1.2V"
io8_166m_hslv_ft_ms_pu_1v2  "IO8_FT 166MHz HSLV med speed @ 1.2V pullup"
io8_166m_hslv_ft_ms_pd_1v2  "IO8_FT 166MHz HSLV med speed @ 1.2V pulldown"
io8_166m_hslv_ft_ls_1v2  "IO8_FT 166MHz HSLV low speed @ 1.2V"
io8_166m_hslv_ft_ls_pu_1v2  "IO8_FT 166MHz HSLV low speed @ 1.2V pullup"
io8_166m_hslv_ft_ls_pd_1v2  "IO8_FT 166MHz HSLV low speed @ 1.2V pulldown"
io8_166m_hslv_ft_hs_1v8  "IO8_FT 166MHz HSLV high speed @ 1.8V"
io8_166m_hslv_ft_hs_pu_1v8  "IO8_FT 166MHz HSLV high speed @ 1.8V pullup"
io8_166m_hslv_ft_hs_pd_1v8  "IO8_FT 166MHz HSLV high speed @ 1.8V pulldown"
io8_166m_hslv_ft_fs_1v8  "IO8_FT 166MHz HSLV fast speed @ 1.8V"
io8_166m_hslv_ft_fs_pu_1v8  "IO8_FT 166MHz HSLV fast speed @ 1.8V pullup"
io8_166m_hslv_ft_fs_pd_1v8  "IO8_FT 166MHz HSLV fast speed @ 1.8V pulldown"
io8_166m_hslv_ft_ms_1v8  "IO8_FT 166MHz HSLV med speed @ 1.8V"
io8_166m_hslv_ft_ms_pu_1v8  "IO8_FT 166MHz HSLV med speed @ 1.8V pullup"
io8_166m_hslv_ft_ms_pd_1v8  "IO8_FT 166MHz HSLV med speed @ 1.8V pulldown"
io8_166m_hslv_ft_ls_1v8  "IO8_FT 166MHz HSLV low speed @ 1.8V"
io8_166m_hslv_ft_ls_pu_1v8  "IO8_FT 166MHz HSLV low speed @ 1.8V pullup"
io8_166m_hslv_ft_ls_pd_1v8  "IO8_FT 166MHz HSLV low speed @ 1.8V pulldown"
io8_166m_hslv_ft_hs_2v5  "IO8_FT 166MHz HSLV high speed @ 2.5V"
io8_166m_hslv_ft_hs_pu_2v5  "IO8_FT 166MHz HSLV high speed @ 2.5V pullup"
io8_166m_hslv_ft_hs_pd_2v5  "IO8_FT 166MHz HSLV high speed @ 2.5V pulldown"
io8_166m_hslv_ft_fs_2v5  "IO8_FT 166MHz HSLV fast speed @ 2.5V"
io8_166m_hslv_ft_fs_pu_2v5  "IO8_FT 166MHz HSLV fast speed @ 2.5V pullup"
io8_166m_hslv_ft_fs_pd_2v5  "IO8_FT 166MHz HSLV fast speed @ 2.5V pulldown"
io8_166m_hslv_ft_ms_2v5  "IO8_FT 166MHz HSLV med speed @ 2.5V"
io8_166m_hslv_ft_ms_pu_2v5  "IO8_FT 166MHz HSLV med speed @ 2.5V pullup"
io8_166m_hslv_ft_ms_pd_2v5  "IO8_FT 166MHz HSLV med speed @ 2.5V pulldown"
io8_166m_hslv_ft_ls_2v5  "IO8_FT 166MHz HSLV low speed @ 2.5V"
io8_166m_hslv_ft_ls_pu_2v5  "IO8_FT 166MHz HSLV low speed @ 2.5V pullup"
io8_166m_hslv_ft_ls_pd_2v5  "IO8_FT 166MHz HSLV low speed @ 2.5V pulldown"
[Model Selector] io8_spi_hslv_ft
io8_spi_ft_hs_1v2  "IO8_FT SPI high speed @ 1.2V"
io8_spi_ft_hs_pu_1v2  "IO8_FT SPI high speed @ 1.2V pullup"
io8_spi_ft_hs_pd_1v2  "IO8_FT SPI high speed @ 1.2V pulldown"
io8_spi_ft_fs_1v2  "IO8_FT SPI fast speed @ 1.2V"
io8_spi_ft_fs_pu_1v2  "IO8_FT SPI fast speed @ 1.2V pullup"
io8_spi_ft_fs_pd_1v2  "IO8_FT SPI fast speed @ 1.2V pulldown"
io8_spi_ft_ms_1v2  "IO8_FT SPI med speed @ 1.2V"
io8_spi_ft_ms_pu_1v2  "IO8_FT SPI med speed @ 1.2V pullup"
io8_spi_ft_ms_pd_1v2  "IO8_FT SPI med speed @ 1.2V pulldown"
io8_spi_ft_ls_1v2  "IO8_FT SPI low speed @ 1.2V"
io8_spi_ft_ls_pu_1v2  "IO8_FT SPI low speed @ 1.2V pullup"
io8_spi_ft_ls_pd_1v2  "IO8_FT SPI low speed @ 1.2V pulldown"
io8_spi_ft_hs_1v8  "IO8_FT SPI high speed @ 1.8V"
io8_spi_ft_hs_pu_1v8  "IO8_FT SPI high speed @ 1.8V pullup"
io8_spi_ft_hs_pd_1v8  "IO8_FT SPI high speed @ 1.8V pulldown"
io8_spi_ft_fs_1v8  "IO8_FT SPI fast speed @ 1.8V"
io8_spi_ft_fs_pu_1v8  "IO8_FT SPI fast speed @ 1.8V pullup"
io8_spi_ft_fs_pd_1v8  "IO8_FT SPI fast speed @ 1.8V pulldown"
io8_spi_ft_ms_1v8  "IO8_FT SPI med speed @ 1.8V"
io8_spi_ft_ms_pu_1v8  "IO8_FT SPI med speed @ 1.8V pullup"
io8_spi_ft_ms_pd_1v8  "IO8_FT SPI med speed @ 1.8V pulldown"
io8_spi_ft_ls_1v8  "IO8_FT SPI low speed @ 1.8V"
io8_spi_ft_ls_pu_1v8  "IO8_FT SPI low speed @ 1.8V pullup"
io8_spi_ft_ls_pd_1v8  "IO8_FT SPI low speed @ 1.8V pulldown"
io8_spi_ft_hs_3v3  "IO8_FT SPI high speed @ 3.3V"
io8_spi_ft_hs_pu_3v3  "IO8_FT SPI high speed @ 3.3V pullup"
io8_spi_ft_hs_pd_3v3  "IO8_FT SPI high speed @ 3.3V pulldown"
io8_spi_ft_fs_3v3  "IO8_FT SPI fast speed @ 3.3V"
io8_spi_ft_fs_pu_3v3  "IO8_FT SPI fast speed @ 3.3V pullup"
io8_spi_ft_fs_pd_3v3  "IO8_FT SPI fast speed @ 3.3V pulldown"
io8_spi_ft_ms_3v3  "IO8_FT SPI med speed @ 3.3V"
io8_spi_ft_ms_pu_3v3  "IO8_FT SPI med speed @ 1.8V pullup"
io8_spi_ft_ms_pd_3v3  "IO8_FT SPI med speed @ 3.3V pulldown"
io8_spi_ft_ls_3v3  "IO8_FT SPI low speed @ 3.3V"
io8_spi_ft_ls_pu_3v3  "IO8_FT SPI low speed @ 3.3V pullup"
io8_spi_ft_ls_pd_3v3  "IO8_FT SPI low speed @ 3.3V pulldown"
io8_spi_hslv_ft_hs_1v2  "IO8_FT SPI HSLV high speed @ 1.2V"
io8_spi_hslv_ft_hs_pu_1v2  "IO8_FT SPI HSLV high speed @ 1.2V pullup"
io8_spi_hslv_ft_hs_pd_1v2  "IO8_FT SPI HSLV high speed @ 1.2V pulldown"
io8_spi_hslv_ft_fs_1v2  "IO8_FT SPI HSLV fast speed @ 1.2V"
io8_spi_hslv_ft_fs_pu_1v2  "IO8_FT SPI HSLV fast speed @ 1.2V pullup"
io8_spi_hslv_ft_fs_pd_1v2  "IO8_FT SPI HSLV fast speed @ 1.2V pulldown"
io8_spi_hslv_ft_ms_1v2  "IO8_FT SPI HSLV med speed @ 1.2V"
io8_spi_hslv_ft_ms_pu_1v2  "IO8_FT SPI HSLV med speed @ 1.2V pullup"
io8_spi_hslv_ft_ms_pd_1v2  "IO8_FT SPI HSLV med speed @ 1.2V pulldown"
io8_spi_hslv_ft_ls_1v2  "IO8_FT SPI HSLV low speed @ 1.2V"
io8_spi_hslv_ft_ls_pu_1v2  "IO8_FT SPI HSLV low speed @ 1.2V pullup"
io8_spi_hslv_ft_ls_pd_1v2  "IO8_FT SPI HSLV low speed @ 1.2V pulldown"
io8_spi_hslv_ft_hs_1v8  "IO8_FT SPI HSLV high speed @ 1.8V"
io8_spi_hslv_ft_hs_pu_1v8  "IO8_FT SPI HSLV high speed @ 1.8V pullup"
io8_spi_hslv_ft_hs_pd_1v8  "IO8_FT SPI HSLV high speed @ 1.8V pulldown"
io8_spi_hslv_ft_fs_1v8  "IO8_FT SPI HSLV fast speed @ 1.8V"
io8_spi_hslv_ft_fs_pu_1v8  "IO8_FT SPI HSLV fast speed @ 1.8V pullup"
io8_spi_hslv_ft_fs_pd_1v8  "IO8_FT SPI HSLV fast speed @ 1.8V pulldown"
io8_spi_hslv_ft_ms_1v8  "IO8_FT SPI HSLV med speed @ 1.8V"
io8_spi_hslv_ft_ms_pu_1v8  "IO8_FT SPI HSLV med speed @ 1.8V pullup"
io8_spi_hslv_ft_ms_pd_1v8  "IO8_FT SPI HSLV med speed @ 1.8V pulldown"
io8_spi_hslv_ft_ls_1v8  "IO8_FT SPI HSLV low speed @ 1.8V"
io8_spi_hslv_ft_ls_pu_1v8  "IO8_FT SPI HSLV low speed @ 1.8V pullup"
io8_spi_hslv_ft_ls_pd_1v8  "IO8_FT SPI HSLV low speed @ 1.8V pulldown"
io8_spi_hslv_ft_hs_2v5  "IO8_FT SPI HSLV high speed @ 2.5V"
io8_spi_hslv_ft_hs_pu_2v5  "IO8_FT SPI HSLV high speed @ 2.5V pullup"
io8_spi_hslv_ft_hs_pd_2v5  "IO8_FT SPI HSLV high speed @ 2.5V pulldown"
io8_spi_hslv_ft_fs_2v5  "IO8_FT SPI HSLV fast speed @ 2.5V"
io8_spi_hslv_ft_fs_pu_2v5  "IO8_FT SPI HSLV fast speed @ 2.5V pullup"
io8_spi_hslv_ft_fs_pd_2v5  "IO8_FT SPI HSLV fast speed @ 2.5V pulldown"
io8_spi_hslv_ft_ms_2v5  "IO8_FT SPI HSLV med speed @ 2.5V"
io8_spi_hslv_ft_ms_pu_2v5  "IO8_FT SPI HSLV med speed @ 2.5V pullup"
io8_spi_hslv_ft_ms_pd_2v5  "IO8_FT SPI HSLV med speed @ 2.5V pulldown"
io8_spi_hslv_ft_ls_2v5  "IO8_FT SPI HSLV low speed @ 2.5V"
io8_spi_hslv_ft_ls_pu_2v5  "IO8_FT SPI HSLV low speed @ 2.5V pullup"
io8_spi_hslv_ft_ls_pd_2v5  "IO8_FT SPI HSLV low speed @ 2.5V pulldown"
[Model Selector] io8_spi_ft
io8_spi_ft_hs_1v2  "IO8_FT SPI high speed @ 1.2V"
io8_spi_ft_hs_pu_1v2  "IO8_FT SPI high speed @ 1.2V pullup"
io8_spi_ft_hs_pd_1v2  "IO8_FT SPI high speed @ 1.2V pulldown"
io8_spi_ft_fs_1v2  "IO8_FT SPI fast speed @ 1.2V"
io8_spi_ft_fs_pu_1v2  "IO8_FT SPI fast speed @ 1.2V pullup"
io8_spi_ft_fs_pd_1v2  "IO8_FT SPI fast speed @ 1.2V pulldown"
io8_spi_ft_ms_1v2  "IO8_FT SPI med speed @ 1.2V"
io8_spi_ft_ms_pu_1v2  "IO8_FT SPI med speed @ 1.2V pullup"
io8_spi_ft_ms_pd_1v2  "IO8_FT SPI med speed @ 1.2V pulldown"
io8_spi_ft_ls_1v2  "IO8_FT SPI low speed @ 1.2V"
io8_spi_ft_ls_pu_1v2  "IO8_FT SPI low speed @ 1.2V pullup"
io8_spi_ft_ls_pd_1v2  "IO8_FT SPI low speed @ 1.2V pulldown"
io8_spi_ft_hs_1v8  "IO8_FT SPI high speed @ 1.8V"
io8_spi_ft_hs_pu_1v8  "IO8_FT SPI high speed @ 1.8V pullup"
io8_spi_ft_hs_pd_1v8  "IO8_FT SPI high speed @ 1.8V pulldown"
io8_spi_ft_fs_1v8  "IO8_FT SPI fast speed @ 1.8V"
io8_spi_ft_fs_pu_1v8  "IO8_FT SPI fast speed @ 1.8V pullup"
io8_spi_ft_fs_pd_1v8  "IO8_FT SPI fast speed @ 1.8V pulldown"
io8_spi_ft_ms_1v8  "IO8_FT SPI med speed @ 1.8V"
io8_spi_ft_ms_pu_1v8  "IO8_FT SPI med speed @ 1.8V pullup"
io8_spi_ft_ms_pd_1v8  "IO8_FT SPI med speed @ 1.8V pulldown"
io8_spi_ft_ls_1v8  "IO8_FT SPI low speed @ 1.8V"
io8_spi_ft_ls_pu_1v8  "IO8_FT SPI low speed @ 1.8V pullup"
io8_spi_ft_ls_pd_1v8  "IO8_FT SPI low speed @ 1.8V pulldown"
io8_spi_ft_hs_3v3  "IO8_FT SPI high speed @ 3.3V"
io8_spi_ft_hs_pu_3v3  "IO8_FT SPI high speed @ 3.3V pullup"
io8_spi_ft_hs_pd_3v3  "IO8_FT SPI high speed @ 3.3V pulldown"
io8_spi_ft_fs_3v3  "IO8_FT SPI fast speed @ 3.3V"
io8_spi_ft_fs_pu_3v3  "IO8_FT SPI fast speed @ 3.3V pullup"
io8_spi_ft_fs_pd_3v3  "IO8_FT SPI fast speed @ 3.3V pulldown"
io8_spi_ft_ms_3v3  "IO8_FT SPI med speed @ 3.3V"
io8_spi_ft_ms_pu_3v3  "IO8_FT SPI med speed @ 1.8V pullup"
io8_spi_ft_ms_pd_3v3  "IO8_FT SPI med speed @ 3.3V pulldown"
io8_spi_ft_ls_3v3  "IO8_FT SPI low speed @ 3.3V"
io8_spi_ft_ls_pu_3v3  "IO8_FT SPI low speed @ 3.3V pullup"
io8_spi_ft_ls_pd_3v3  "IO8_FT SPI low speed @ 3.3V pulldown"
io8_spi_hslv_ft_hs_1v2  "IO8_FT SPI HSLV high speed @ 1.2V"
io8_spi_hslv_ft_hs_pu_1v2  "IO8_FT SPI HSLV high speed @ 1.2V pullup"
io8_spi_hslv_ft_hs_pd_1v2  "IO8_FT SPI HSLV high speed @ 1.2V pulldown"
io8_spi_hslv_ft_fs_1v2  "IO8_FT SPI HSLV fast speed @ 1.2V"
io8_spi_hslv_ft_fs_pu_1v2  "IO8_FT SPI HSLV fast speed @ 1.2V pullup"
io8_spi_hslv_ft_fs_pd_1v2  "IO8_FT SPI HSLV fast speed @ 1.2V pulldown"
io8_spi_hslv_ft_ms_1v2  "IO8_FT SPI HSLV med speed @ 1.2V"
io8_spi_hslv_ft_ms_pu_1v2  "IO8_FT SPI HSLV med speed @ 1.2V pullup"
io8_spi_hslv_ft_ms_pd_1v2  "IO8_FT SPI HSLV med speed @ 1.2V pulldown"
io8_spi_hslv_ft_ls_1v2  "IO8_FT SPI HSLV low speed @ 1.2V"
io8_spi_hslv_ft_ls_pu_1v2  "IO8_FT SPI HSLV low speed @ 1.2V pullup"
io8_spi_hslv_ft_ls_pd_1v2  "IO8_FT SPI HSLV low speed @ 1.2V pulldown"
io8_spi_hslv_ft_hs_1v8  "IO8_FT SPI HSLV high speed @ 1.8V"
io8_spi_hslv_ft_hs_pu_1v8  "IO8_FT SPI HSLV high speed @ 1.8V pullup"
io8_spi_hslv_ft_hs_pd_1v8  "IO8_FT SPI HSLV high speed @ 1.8V pulldown"
io8_spi_hslv_ft_fs_1v8  "IO8_FT SPI HSLV fast speed @ 1.8V"
io8_spi_hslv_ft_fs_pu_1v8  "IO8_FT SPI HSLV fast speed @ 1.8V pullup"
io8_spi_hslv_ft_fs_pd_1v8  "IO8_FT SPI HSLV fast speed @ 1.8V pulldown"
io8_spi_hslv_ft_ms_1v8  "IO8_FT SPI HSLV med speed @ 1.8V"
io8_spi_hslv_ft_ms_pu_1v8  "IO8_FT SPI HSLV med speed @ 1.8V pullup"
io8_spi_hslv_ft_ms_pd_1v8  "IO8_FT SPI HSLV med speed @ 1.8V pulldown"
io8_spi_hslv_ft_ls_1v8  "IO8_FT SPI HSLV low speed @ 1.8V"
io8_spi_hslv_ft_ls_pu_1v8  "IO8_FT SPI HSLV low speed @ 1.8V pullup"
io8_spi_hslv_ft_ls_pd_1v8  "IO8_FT SPI HSLV low speed @ 1.8V pulldown"
io8_spi_hslv_ft_hs_2v5  "IO8_FT SPI HSLV high speed @ 2.5V"
io8_spi_hslv_ft_hs_pu_2v5  "IO8_FT SPI HSLV high speed @ 2.5V pullup"
io8_spi_hslv_ft_hs_pd_2v5  "IO8_FT SPI HSLV high speed @ 2.5V pulldown"
io8_spi_hslv_ft_fs_2v5  "IO8_FT SPI HSLV fast speed @ 2.5V"
io8_spi_hslv_ft_fs_pu_2v5  "IO8_FT SPI HSLV fast speed @ 2.5V pullup"
io8_spi_hslv_ft_fs_pd_2v5  "IO8_FT SPI HSLV fast speed @ 2.5V pulldown"
io8_spi_hslv_ft_ms_2v5  "IO8_FT SPI HSLV med speed @ 2.5V"
io8_spi_hslv_ft_ms_pu_2v5  "IO8_FT SPI HSLV med speed @ 2.5V pullup"
io8_spi_hslv_ft_ms_pd_2v5  "IO8_FT SPI HSLV med speed @ 2.5V pulldown"
io8_spi_hslv_ft_ls_2v5  "IO8_FT SPI HSLV low speed @ 2.5V"
io8_spi_hslv_ft_ls_pu_2v5  "IO8_FT SPI HSLV low speed @ 2.5V pullup"
io8_spi_hslv_ft_ls_pd_2v5  "IO8_FT SPI HSLV low speed @ 2.5V pulldown"
[Define Package Model]  481-wlcsp-150-1rdl-nodsi-220909
[Manufacturer]  Unknown
[OEM]  Unknown
[Description]  None
[Number Of Pins]  149
[Pin Numbers]
| Pin Num   Terminal Name
T12 | NRST
T10 | PA0
W11 | PA1
R9 | PA2
V10 | PA3
P8 | PA4
AA11 | PA5
U9 | PA6
Y10 | PA7
G3 | PA8
F2 | PA9
E3 | PA10
E1 | PA11
C1 | PA12
D2 | PA13
H4 | PA14
F4 | PA15
T8 | PB0
W9 | PB1
AB10 | PB2
K8 | PB3
L9 | PB4
A9 | PB5
E9 | PB6
C9 | PB7
J9 | PB8
B10 | PB9
W3 | PB10
AA3 | PB11
Y2 | PB12
R5 | PB13
T4 | PB14
N5 | PB15
N9 | PC0
M8 | PC1
V12 | PC2
U11 | PC3
AC11 | PC4
N7 | PC5
J3 | PC6
L5 | PC7
G1 | PC8
H2 | PC9
D4 | PC10
B4 | PC11
J5 | PC12
D12 | PC13
E13 | PC14-OSC32_IN
G13 | PC15-OSC32_OUT
G5 | PD0
E5 | PD1
C5 | PD2
A5 | PD3
H6 | PD4
F6 | PD5
K6 | PD6
L7 | PD7
W1 | PD8
V2 | PD9
U3 | PD10
P4 | PD11
R3 | PD12
U1 | PD13
N3 | PD14
P2 | PD15
M10 | PE0
K10 | PE1
A13 | PE2
D10 | PE3
F10 | PE4
H10 | PE5
E11 | PE6
AB8 | PE7
V6 | PE8
U5 | PE9
Y6 | PE10
W5 | PE11
V4 | PE12
Y4 | PE13
AB6 | PE14
AA5 | PE15
G11 | PF0
H12 | PF1
J13 | PF2
K12 | PF3
J11 | PF4
L11 | PF5
N11 | PF6
N13 | PF7
P10 | PF8
P12 | PF9
R11 | PF10
R7 | PF11
V8 | PF12
P6 | PF13
U7 | PF14
Y8 | PF15
T6 | PG0
W7 | PG1
N1 | PG2
M4 | PG3
M2 | PG4
L3 | PG5
M6 | PG6
L1 | PG7
K4 | PG8
J7 | PG9
E7 | PG10
C7 | PG11
A7 | PG12
G7 | PG13
F8 | PG14
H8 | PG15
R13 | PH0-OSC_IN
U13 | PH1-OSC_OUT
G9 | PH3-BOOT0
AB2 | VDD11
A11 | VDD11
B2 | VDD11
C13 | VBAT
A1 | VDDUSB
A3 | VDD
AB12 | VDD
AC1 | VDD
AC7 | VDD
AC9 | VDD
B6 | VDD
B12 | VDD
L13 | VDD
R1 | VDD
AA13 | VDDA
J1 | VDDIO2
B8 | VDDIO2
AB4 | VDDSMPS
AC5 | VLXSMPS
Y12 | VREFP
AA1 | VSS
AA7 | VSS
AA9 | VSS
AC13 | VSS
C3 | VSS
C11 | VSS
D6 | VSS
D8 | VSS
K2 | VSS
F12 | VSS
T2 | VSS
W13 | VSSA_VREFM
AC3 | VSSSMPS
|[Merged Pins]  F12
|M12  |  VSS
[Model Data]
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[End Model Data]
[End Package Model]
| Models and submodels in the file (265): io8_100m_ft_hs_1v2 (I/O), io8_100m_ft_hs_pu_1v2 (I/O), io8_100m_ft_hs_pd_1v2 (I/O), io8_100m_ft_fs_1v2 (I/O), io8_100m_ft_fs_pu_1v2 (I/O), io8_100m_ft_fs_pd_1v2 (I/O), io8_100m_ft_ms_1v2 (I/O), io8_100m_ft_ms_pu_1v2 (I/O), io8_100m_ft_ms_pd_1v2 (I/O), io8_100m_ft_ls_1v2 (I/O), io8_100m_ft_ls_pu_1v2 (I/O), io8_100m_ft_ls_pd_1v2 (I/O), io8_100m_ft_hs_1v8 (I/O), io8_100m_ft_hs_pu_1v8 (I/O), io8_100m_ft_hs_pd_1v8 (I/O), io8_100m_ft_fs_1v8 (I/O), io8_100m_ft_fs_pu_1v8 (I/O), io8_100m_ft_fs_pd_1v8 (I/O), io8_100m_ft_ms_1v8 (I/O), io8_100m_ft_ms_pu_1v8 (I/O), io8_100m_ft_ms_pd_1v8 (I/O), io8_100m_ft_ls_1v8 (I/O), io8_100m_ft_ls_pu_1v8 (I/O), io8_100m_ft_ls_pd_1v8 (I/O), io8_100m_ft_hs_3v3 (I/O), io8_100m_ft_hs_pu_3v3 (I/O), io8_100m_ft_hs_pd_3v3 (I/O), io8_100m_ft_fs_3v3 (I/O), io8_100m_ft_fs_pu_3v3 (I/O), io8_100m_ft_fs_pd_3v3 (I/O), io8_100m_ft_ms_3v3 (I/O), io8_100m_ft_ms_pu_3v3 (I/O), io8_100m_ft_ms_pd_3v3 (I/O), io8_100m_ft_ls_3v3 (I/O), io8_100m_ft_ls_pu_3v3 (I/O), io8_100m_ft_ls_pd_3v3 (I/O), io8_100m_hslv_ft_hs_1v2 (I/O), io8_100m_hslv_ft_hs_pu_1v2 (I/O), io8_100m_hslv_ft_hs_pd_1v2 (I/O), io8_100m_hslv_ft_fs_1v2 (I/O), io8_100m_hslv_ft_fs_pu_1v2 (I/O), io8_100m_hslv_ft_fs_pd_1v2 (I/O), io8_100m_hslv_ft_ms_1v2 (I/O), io8_100m_hslv_ft_ms_pu_1v2 (I/O), io8_100m_hslv_ft_ms_pd_1v2 (I/O), io8_100m_hslv_ft_ls_1v2 (I/O), io8_100m_hslv_ft_ls_pu_1v2 (I/O), io8_100m_hslv_ft_ls_pd_1v2 (I/O), io8_100m_hslv_ft_hs_1v8 (I/O), io8_100m_hslv_ft_hs_pu_1v8 (I/O), io8_100m_hslv_ft_hs_pd_1v8 (I/O), io8_100m_hslv_ft_fs_1v8 (I/O), io8_100m_hslv_ft_fs_pu_1v8 (I/O), io8_100m_hslv_ft_fs_pd_1v8 (I/O), io8_100m_hslv_ft_ms_1v8 (I/O), io8_100m_hslv_ft_ms_pu_1v8 (I/O), io8_100m_hslv_ft_ms_pd_1v8 (I/O), io8_100m_hslv_ft_ls_1v8 (I/O), io8_100m_hslv_ft_ls_pu_1v8 (I/O), io8_100m_hslv_ft_ls_pd_1v8 (I/O), io8_100m_hslv_ft_hs_2v5 (I/O), io8_100m_hslv_ft_hs_pu_2v5 (I/O), io8_100m_hslv_ft_hs_pd_2v5 (I/O), io8_100m_hslv_ft_fs_2v5 (I/O), io8_100m_hslv_ft_fs_pu_2v5 (I/O), io8_100m_hslv_ft_fs_pd_2v5 (I/O), io8_100m_hslv_ft_ms_2v5 (I/O), io8_100m_hslv_ft_ms_pu_2v5 (I/O), io8_100m_hslv_ft_ms_pd_2v5 (I/O), io8_100m_hslv_ft_ls_2v5 (I/O), io8_100m_hslv_ft_ls_pu_2v5 (I/O), io8_100m_hslv_ft_ls_pd_2v5 (I/O), io8_100m_i2c_ft_1v2 (I/O_open_drain), io8_100m_i2c_ft_pu_1v2 (I/O_open_drain), io8_100m_i2c_ft_pd_1v2 (I/O_open_drain), io8_100m_i2c_ft_1v8 (I/O_open_drain), io8_100m_i2c_ft_pu_1v8 (I/O_open_drain), io8_100m_i2c_ft_pd_1v8 (I/O_open_drain), io8_100m_i2c_ft_3v3 (I/O_open_drain), io8_100m_i2c_ft_pu_3v3 (I/O_open_drain)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
